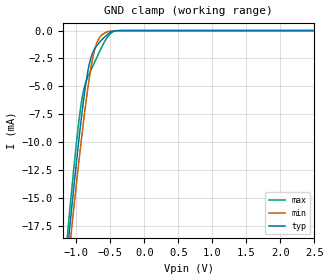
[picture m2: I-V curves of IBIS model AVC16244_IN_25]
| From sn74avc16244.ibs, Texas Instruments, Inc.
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[Model]   AVC16244_IN_25
Model_type  Input
Vinl=0.7
Vinh=1.7
| variable   typ   min   max
C_comp   4.38pF   3.10pF   5.84pF
[Temperature Range]   40   100   -40
| Ambient temperature   25   85   -40
[Voltage range]   2.5   2.3   2.7
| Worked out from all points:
|   GND clamp passes 1 mA (typ) near -0.65 V on its own axis
[GND Clamp]
| AVC16244_IN_25
|   Voltage   I(typ)   I(min)   I(max)
-2.5V     -112.3mA   -109.5mA   -117.9mA
-1.135V   -19.96mA   -21.59mA   -18.58mA
-1.1V     -17.8mA    -19.52mA   -16.29mA
-1.07V    -15.97mA   -17.77mA   -14.36mA
-935mV    -8.266mA   -10.23mA   -6.794mA
-885mV    -5.803mA   -7.664mA   -5.121mA
-825mV    -3.453mA   -4.886mA   -4.059mA
-715mV    -1.486mA   -1.371mA   -2.62mA
-595mV    -633.2uA   -258.5uA   -1.097mA
-485mV    -114.6uA   -32.39uA   -203.1uA
-380mV    -5.569uA   -5.168uA   -5.667uA
2.5V      211.4pA    710.6pA    13.87pA
